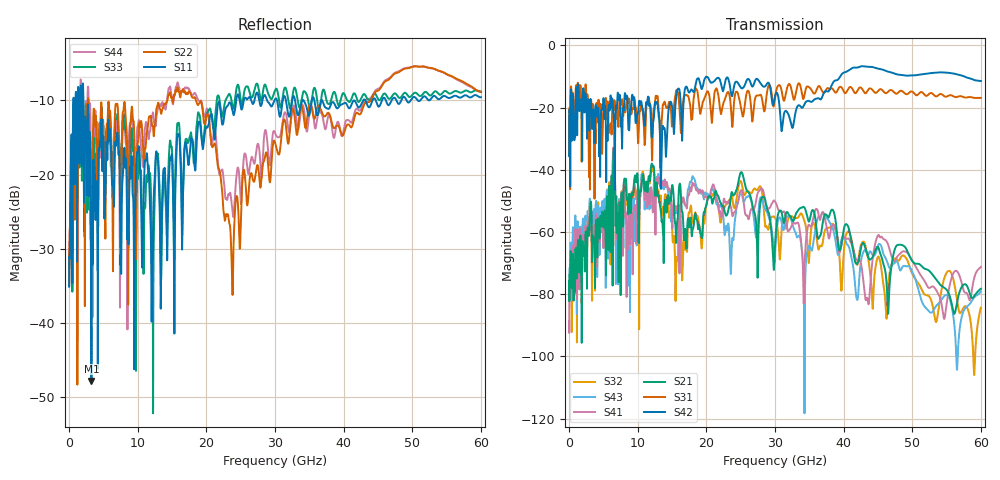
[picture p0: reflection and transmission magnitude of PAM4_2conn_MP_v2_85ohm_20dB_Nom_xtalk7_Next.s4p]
! Info: Touchstone file created by Circ.  Input file=FAB50GbE_2conn_Midplane_Examax_Topo2_v2_85ohm_20dB_Nom.circ
# Hz S RI R 50
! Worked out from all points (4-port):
!   6000 points, 10 MHz to 60 GHz, reference 50 ohm
!   strongest paths, dB at 10 MHz, 15.01 GHz, 30.01 GHz, 45.01 GHz, 60 GHz:
!     S42: -35.6, -19.6, -16.3, -7.5, -11.4
!     S31: -35.4, -26.0, -16.8, -14.6, -16.9
!     S21: -75.7, -45.1, -64.3, -64.8, -78.3
!     S41: -88.7, -57.5, -50.2, -61.1, -71.2
!     S43: -77.4, -53.6, -67.1, -64.5, -79.2
!     S32: -81.8, -57.5, -55.4, -68.0, -84.3
!   lowest |S11| = -47.8 dB at 3.26 GHz (marker M1), VSWR 1.01, Z = 50.3 - j0.266 ohm
!   |S11| at or under -10 dB: 2.089 GHz to 24.35 GHz (22.26 GHz wide, 168 % of centre); 36.89 GHz to 41.5 GHz (4.614 GHz wide, 11.8 % of centre); 41.56 GHz to 42.85 GHz (1.293 GHz wide, 3.06 % of centre)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
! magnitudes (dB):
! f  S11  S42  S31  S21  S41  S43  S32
! 10 MHz  -35.1  -35.6  -35.4  -75.7  -88.7  -77.4  -81.8
! 3.26 GHz  -47.8  -20.2  -18.8  -53.7  -59.7  -56.1  -60.0
! 15.61 GHz  -18.3  -16.7  -14.5  -63.5  -51.7  -53.9  -71.8
! 25.11 GHz  -11.2  -13.8  -20.9  -40.7  -46.5  -47.3  -44.0
! 29.79 GHz  -10.3  -18.7  -19.7  -71.0  -49.9  -65.5  -54.9
! 43.36 GHz  -10.4  -6.8  -15.0  -66.5  -81.3  -66.7  -66.4
! 60 GHz  -9.6  -11.4  -16.9  -78.3  -71.2  -79.2  -84.3
